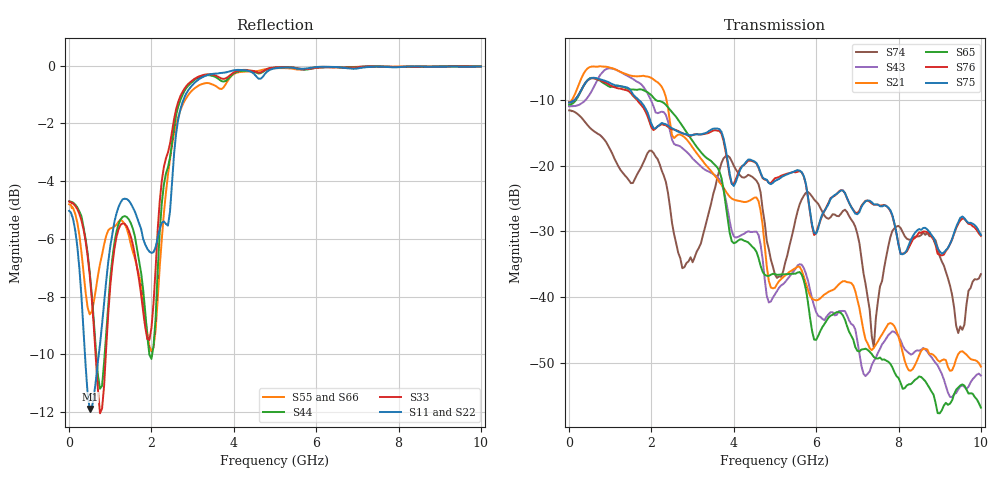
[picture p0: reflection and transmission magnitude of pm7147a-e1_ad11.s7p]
# GHz S DB R 50
! S-Parameters data
! Freq  dbS11  angS11  dbS12  angS12  dbS13  angS13  dbS14  angS14
!  dbS15  angS15  dbS16  angS16  dbS17  angS17  dbS21  angS21
!  dbS22  angS22  dbS23  angS23  dbS24  angS24  dbS25  angS25
!  dbS26  angS26  dbS27  angS27  dbS31  angS31  dbS32  angS32
!  dbS33  angS33  dbS34  angS34  dbS35  angS35  dbS36  angS36
!  dbS37  angS37  dbS41  angS41  dbS42  angS42  dbS43  angS43
!  dbS44  angS44  dbS45  angS45  dbS46  angS46  dbS47  angS47
!  dbS51  angS51  dbS52  angS52  dbS53  angS53  dbS54  angS54
!  dbS55  angS55  dbS56  angS56  dbS57  angS57  dbS61  angS61
!  dbS62  angS62  dbS63  angS63  dbS64  angS64  dbS65  angS65
!  dbS66  angS66  dbS67  angS67  dbS71  angS71  dbS72  angS72
!  dbS73  angS73  dbS74  angS74  dbS75  angS75  dbS76  angS76
!  dbS77  angS77
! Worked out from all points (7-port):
!   279 points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, 1 Hz to 10 GHz, reference 50 ohm
!   strongest paths, dB at 1 Hz, 7.943 MHz, 3.05 GHz, 6.55 GHz, 10 GHz:
!     S75: -10.4, -10.4, -15.3, -24.0, -30.5
!     S76: -10.4, -10.4, -15.2, -23.9, -30.7
!     S65: -10.7, -10.7, -16.7, -42.3, -56.8
!     S21: -10.3, -10.3, -17.7, -38.1, -50.6
!     S43: -11.0, -11.0, -19.2, -42.1, -51.9
!     S74: -11.6, -11.6, -33.9, -27.7, -36.5
!   lowest |S11| = -11.9 dB at 500 MHz (marker M1), VSWR 1.68, Z = 29.8 + j1.38 ohm
!   |S11| at or under -10 dB: 384.6 MHz to 721.5 MHz (336.9 MHz wide, 60.9 % of centre)
